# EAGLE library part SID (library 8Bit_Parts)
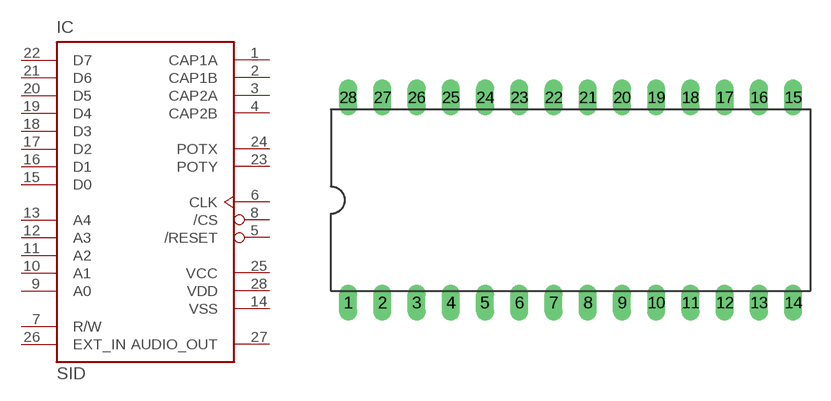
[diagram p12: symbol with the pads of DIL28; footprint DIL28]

Designator prefix IC

## SID  [DIL28]
1  CAP1A  in
2  CAP1B  in
3  CAP2A  in
4  CAP2B  in
5  /RESET  in
6  CLK  in
7  R/W  in
8  /CS  in
9  A0  in
10  A1  in
11  A2  in
12  A3  in
13  A4  in
14  VSS  pwr
15  D0
16  D1
17  D2
18  D3
19  D4
20  D5
21  D6
22  D7
23  POTY  in
24  POTX  in
25  VCC  pwr
26  EXT_IN  in
27  AUDIO_OUT  out
28  VDD  pwr

## Footprint DIL28 (pad centres in mm)
Dual In Line Package
drill 0.813 long: 1 -16.51,-7.62; 2 -13.97,-7.62; 3 -11.43,-7.62; 4 -8.89,-7.62; 5 -6.35,-7.62; 6 -3.81,-7.62; 7 -1.27,-7.62; 8 1.27,-7.62; 9 3.81,-7.62; 10 6.35,-7.62; 11 8.89,-7.62; 12 11.43,-7.62; 13 13.97,-7.62; 14 16.51,-7.62; 15 16.51,7.62; 16 13.97,7.62; 17 11.43,7.62; 18 8.89,7.62; 19 6.35,7.62; 20 3.81,7.62; 21 1.27,7.62; 22 -1.27,7.62; 23 -3.81,7.62; 24 -6.35,7.62; 25 -8.89,7.62; 26 -11.43,7.62; 27 -13.97,7.62; 28 -16.51,7.62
